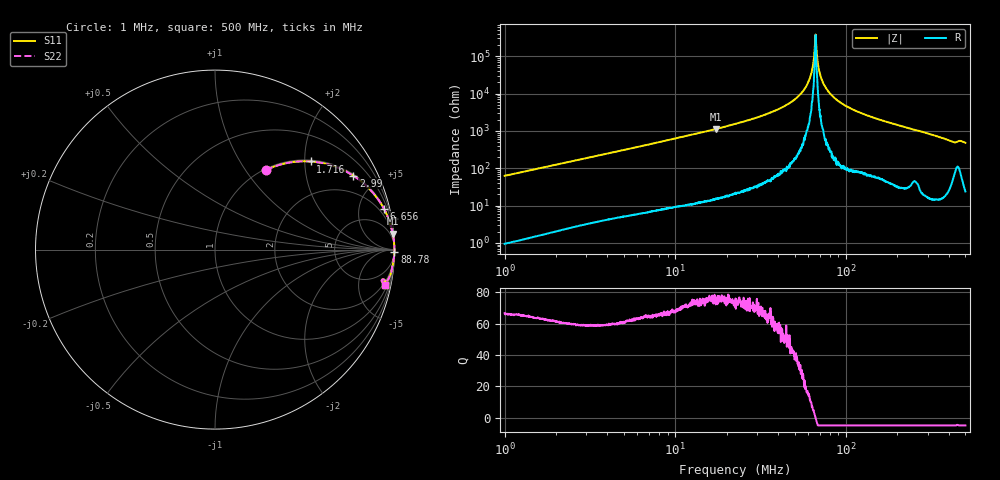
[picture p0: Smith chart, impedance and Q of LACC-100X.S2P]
!s-Parameter Generated by FASTRON Sdn. Bhd.
!FASTRON P/N : LACC-100X
!Keysight Technologies,E4991B,MY54100416,A.01.15
!Date: Wed Mar 18 09:26:33 2026
!Version  : Rev00 Wed Mar 18 09:26:33 2026
!Data & Calibration Information:
!PortZ  Port1:50+j0  Port2:50+j0
!When reading, reference impedance value at option line is always used.
!Remarks : This data is being provided solely for informational purposes.
!Freq	S11	S21	S12	S22
# Hz S dB R 50
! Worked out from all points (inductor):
!   1601 points, 1 MHz to 500 MHz, reference 50 ohm
!   read as one part in series: L = 9.92 uH near 1.032 MHz
!   highest Q = 76.5 at 17.24 MHz (marker M1), where L = 10.4 uH
!   self-resonance near 66.09 MHz
!   S11 on the Smith chart (normalised r, x): 1 MHz: 1.02, +1.25; 1.716 MHz: 1.03, +2.14; 2.99 MHz: 1.06, +3.70; 6.656 MHz: 1.13, +8.23; 88.78 MHz: open; 500 MHz: 1.48, -9.62
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1000000  -5.58 57.4  -1.49 -31.7  -1.49 -31.7  -5.58 57.4
1715825  -2.80 42.7  -3.37 -46.4  -3.37 -46.4  -2.80 42.7
2820919  -1.29 29.5  -6.14 -59.5  -6.14 -59.5  -1.29 29.5
2990153  -1.17 28.1  -6.53 -60.9  -6.53 -60.9  -1.17 28.1
6655579  -0.28 13.6  -12.57 -75.5  -12.57 -75.5  -0.28 13.6
7957584  -0.20 11.4  -14.06 -77.7  -14.06 -77.7  -0.20 11.4
1.723716e7  -0.04 5.1  -21.06 -84.1  -21.06 -84.1  -0.04 5.1
2.236068e7  -0.03 3.7  -23.71 -85.5  -23.71 -85.5  -0.03 3.7
3.563754e7  -0.01 1.9  -29.62 -87.2  -29.62 -87.2  -0.01 1.9
4.824836e7  -0.00 0.9  -35.80 -87.7  -35.80 -87.7  -0.00 0.9
5.746337e7  -0.00 0.4  -42.85 -86.5  -42.85 -86.5  -0.00 0.4
6.067462e7  -0.00 0.3  -47.06 -85.9  -47.06 -85.9  -0.00 0.3
6.307767e7  -0.00 0.1  -52.10 -81.3  -52.10 -81.3  -0.00 0.1
6.506845e7  -0.00 0.1  -60.21 -71.8  -60.21 -71.8  -0.00 0.1
6.660267e7  -0.00 -0.0  -68.64 35.1  -68.64 35.1  -0.00 -0.0
6.790877e7  -0.00 -0.1  -58.19 75.8  -58.19 75.8  -0.00 -0.1
7.032465e7  -0.00 -0.2  -50.48 85.5  -50.48 85.5  -0.00 -0.2
7.339442e7  -0.00 -0.3  -45.70 86.5  -45.70 86.5  -0.00 -0.3
8.878078e7  -0.00 -0.9  -36.42 87.8  -36.42 87.8  -0.00 -0.9
1.156179e8  -0.01 -1.7  -30.48 86.9  -30.48 86.9  -0.01 -1.7
1.77937e8  -0.03 -3.4  -24.54 85.2  -24.54 85.2  -0.03 -3.4
5e8  -0.27 -11.6  -13.92 75.6  -13.92 75.6  -0.27 -11.6
